ORGANIZATION_BLOCK MAIN:OB1
TITLE=Gestione Garage automatico
//Simulatore: 11
//Versione: 1.0
//Data: 28/02/2002
//----------- Descrizione dell'impianto------------------
//In un garage, l'entrata e l'uscita sono regolate da due
//sbarre. Ambedue le sbarre vengono chiuse e aperte tramite
//un motore (rispettivamente M1 e M2).
//Prima di ogni sbarra è installato un sensore di prossimità
//(entrata SQ1, uscita SQ4) che rileva la presenza del veicolo.
//Immediatamente dopo ogni sbarra è installato un fotosensore
//(entrata B1, uscita B2) atte a rilevare il passaggio del
//veivolo.
//------ Entrata autoveicoli ----------------------------
//Se viene attivato il sensore SQ1 dalla presenza di un
//veicolo entrate immediatamente dopo aver premuto il pulsante
//SB1 per il ritiro del talloncino di ingresso, la sbarra di
//entrata viene aperta tramite il motore M1. Quando il mezzo ha
//superato il fotosensore B1, il motore M1 richiude la sbarra.
//Contemporaneamente il contatore viene incrementato di una
//unità. Quando nel garage sono presenti 6 veicoli la sbarra
//d'entrata viene bloccata e il semaforo in entrata diventa
//rosso. Per il corretto funzionamento del motore M1, la
//posizione della sbarra viene rilevata tramite due finecorsa
//SQ2 (sbarra chiusa) e SQ3 (sbarra aperta).
//------ Uscita autoveicoli ----------------------------
//Quando il veicolo in uscita attiva il sensore SQ4 subito
//dopo aver premuto il pulsante SB2, che simula il pagamento
//del pedaggio, il semaforo in uscita passa al verde e la
//sbarra viene aperta dal motore M2.
//Quando il mezzo ha superato il fotosensore B2 il motore
//M2 richiude la sbarra e il semaforo passa al rosso; nello
//stesso tempo il contatore viene decrementato di un'unità
//e viene così gestita in modo automatico l'occupazione del
//garage.
//Per il corretto funzionamento del motore M1 la
//posizione della sbarra viene rilevata tramite due finecorsa
//SQ5 (sbarra chiusa) e SQ6 (sbarra aperta).
//
//L'azionamento delle sbarre viene anche segnalato dal
//lampeggio di due lampade HL5( entrata) HL6 (uscita).
//I motori che azionano le sbarre sono protetti da due
//relè termici FR1 e FR2. In caso di intervento la
//sequenza interrotta potrà essere completata azionando
//il relativo pulsante.

BEGIN
NETWORK 1 //Reset merker memoria chiusura sbarre
//
LD SM0.1
R M0.0 2

NETWORK 2 //Apertura sbarra ingresso
//
LDN C0
AN M0.0
A I0.1
A I0.0
O Q0.0
AN I0.6
A I0.7
A I0.3
= Q0.0

NETWORK 3 //Set merker memoria chiusura sbarra ingresso
//
LD I0.4
S M0.0 1

NETWORK 4 //Reset merker memoria chiusura sbarra ingresso
//
LDN I0.2
R M0.0 1

NETWORK 5 //Chiusura sbarra ingresso
//
LD I0.0
A M0.0
O I0.4
O Q0.1
A I0.2
A I0.7
AN I0.5
= Q0.1

NETWORK 6 //Contatore Auto
//
LD I0.4
LD I1.4
LD SM0.1
CTUD C0 +6

NETWORK 7 //Apertura sbarra Uscita
//
LD I1.1
AN M0.1
A I1.0
O Q0.7
AN I1.5
A I1.7
A I1.3
= Q0.7

NETWORK 8 //Set merker memoria chiusura sbarra uscita
//
LD I1.4
ED
S M0.1 1

NETWORK 9 //Reset merker memoria chiusura sbarra uscita
//
LDN I1.2
R M0.1 1

NETWORK 10 //Chiusura sbarra Uscita
//
LD I1.4
ED
LD I1.0
A M0.1
OLD
O Q0.6
AN I1.6
A I1.7
A I1.2
= Q0.6

NETWORK 11 //Lampeggio ingresso
//
LD I0.2
A SM0.5
= Q1.0

NETWORK 12 //Lampeggio Uscita
//
LD I1.2
A SM0.5
= Q1.1

NETWORK 13 //Abilita Semaforo rosso in ingresso
//
LD C0
= Q0.3

NETWORK 14 //Abilita Semaforo verde in ingresso
//
LDN C0
= Q0.2

NETWORK 15 //Abilita semaforo verde in uscita
//
LDN I1.3
= Q0.4

NETWORK 16 //Abilita semaforo Rosso in uscita
//
LD I1.3
= Q0.5

END_ORGANIZATION_BLOCK

